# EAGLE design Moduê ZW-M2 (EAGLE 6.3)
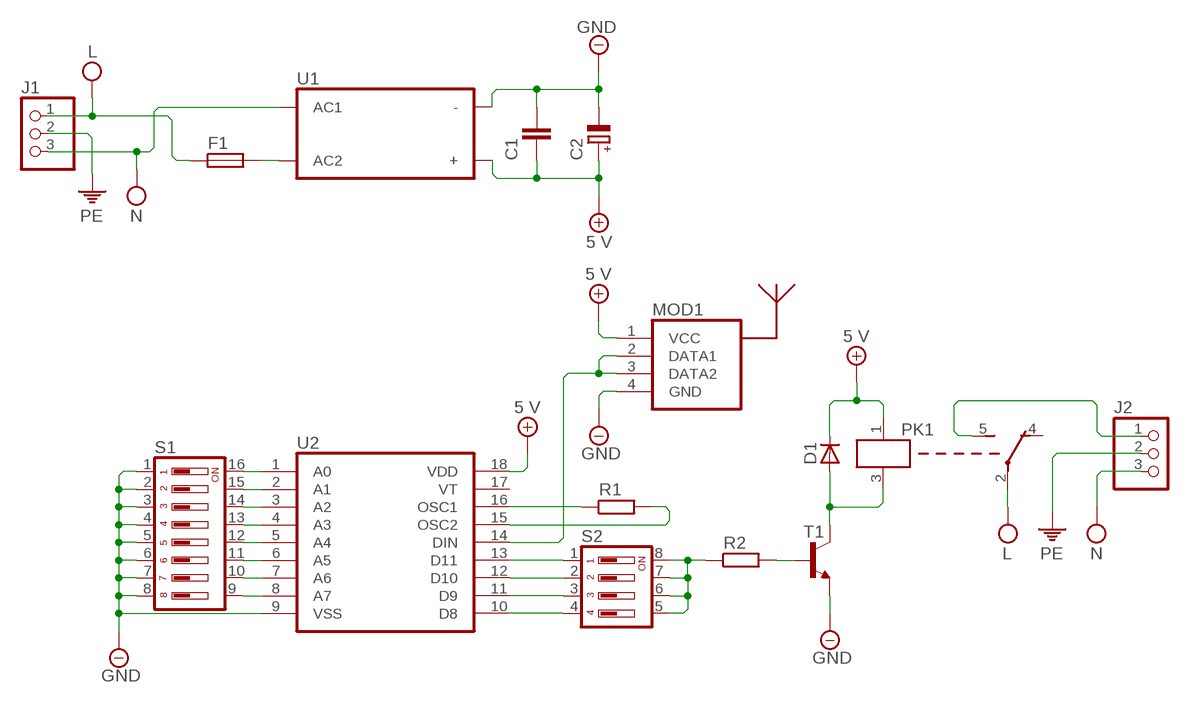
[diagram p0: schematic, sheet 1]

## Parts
C1  KONDENSATOR_CERAMICZNY  [KONDENSATOR_CERAMICZNY]
C2  KONDENSATOR_ELEKTROLITYCZNY_1  [KONDENSATOR_ELEKTROLITYCZNY_1]
D1  DIODA_PROSTOWNICZA  [DIODA_PROSTOWNICZA]
F1  BEZPIECZNIK  [BEZPIECZNIK]
J1  ZLACZE_230V  [ZLACZE_230V]
J2  ZLACZE_230V  [ZLACZE_230V]
MOD1  ODBIORNIK433MHZ  [ODBIORNIK433MHZ]
PK1  PRZEKAZNIK  [PRZEKAZNIK]
R1  REZYSTOR  [REZYSTOR]
R2  REZYSTOR  [REZYSTOR]
S1  DIP_SWITCH_8  [DIP_SWITCH_8]
S2  DIP_SWITCH_4  [DIP_SWITCH_4]
T1  TRANZYSTOR_2N3904  [TRANZYSTOR_2N3904]
U1  ZASILACZ  [ZASILACZ]
U2  HT12D  [HT12D]

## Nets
5V: C1.2 C2.+ D1.C MOD1.1(VCC) PK1.1(A1) U1.+ U2.18(VDD) ; supply symbol labelled 5 V
GND: C1.1 C2.- MOD1.4(GND) S1.1 S1.2 S1.3 S1.4 S1.5 S1.6 S1.7 S1.8 T1.E U1.- U2.9(VSS)
L: F1.1 J1.1 PK1.2(C)
N: J1.3 J2.3 U1.AC1
N$1: F1.2 U1.AC2
N$2: J2.1 PK1.5(NO)
N$3: S2.1 U2.13(D11)
N$4: S2.2 U2.12(D10)
N$5: S2.3 U2.11(D9)
N$6: S2.4 U2.10(D8)
N$7: S1.9 U2.8(A7)
N$8: R2.2 T1.B
N$9: R2.1 S2.5 S2.6 S2.7 S2.8
N$10: S1.10 U2.7(A6)
N$11: S1.11 U2.6(A5)
N$12: S1.12 U2.5(A4)
N$13: S1.13 U2.4(A3)
N$14: S1.14 U2.3(A2)
N$15: S1.15 U2.2(A1)
N$16: S1.16 U2.1(A0)
N$17: MOD1.2(DATA1) MOD1.3(DATA2) U2.14(DIN)
N$20: D1.A PK1.3(A2) T1.C
N$29: R1.2 U2.15(OSC2)
N$30: R1.1 U2.16(OSC1)
PE: J1.2 J2.2
Unconnected: PK1.4(NC) U2.17(VT)

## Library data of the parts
C1 = Własne:KONDENSATOR_CERAMICZNY
C2 = Własne:KONDENSATOR_ELEKTROLITYCZNY_1
D1 = Własne:DIODA_PROSTOWNICZA
F1 = Własne:BEZPIECZNIK
J1 J2 = Moje:ZLACZE_230V
MOD1 = Własne:ODBIORNIK433MHZ
PK1 = Moje:PRZEKAZNIK
R1 R2 = Własne:REZYSTOR
S1 = Własne:DIP_SWITCH_8
S2 = Własne:DIP_SWITCH_4
T1 = Własne:TRANZYSTOR_2N3904
U1 = Własne:ZASILACZ
U2 = Własne:HT12D

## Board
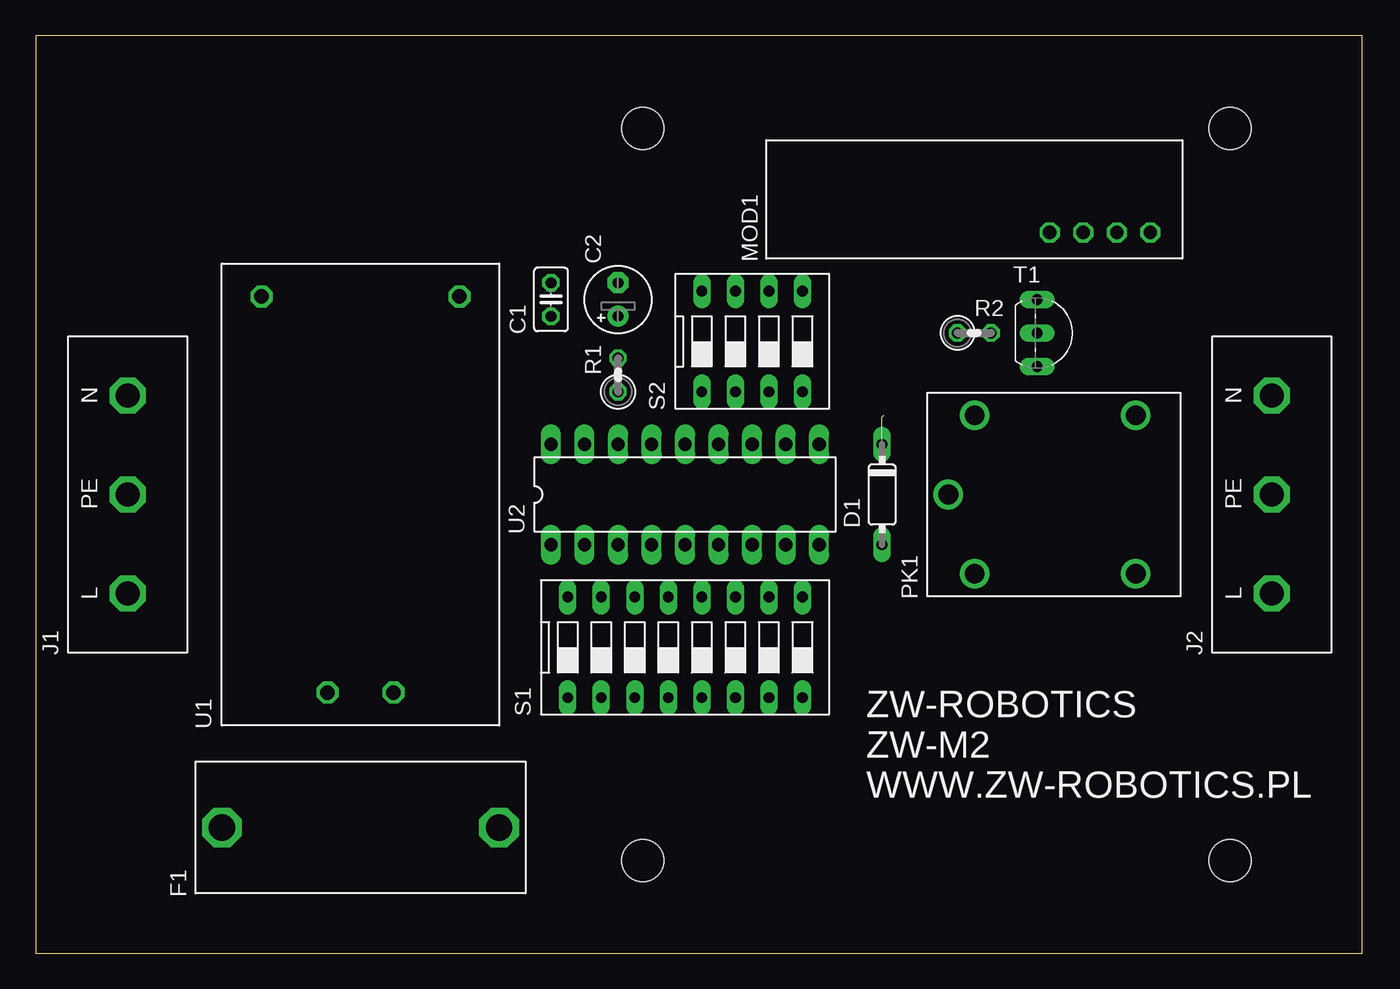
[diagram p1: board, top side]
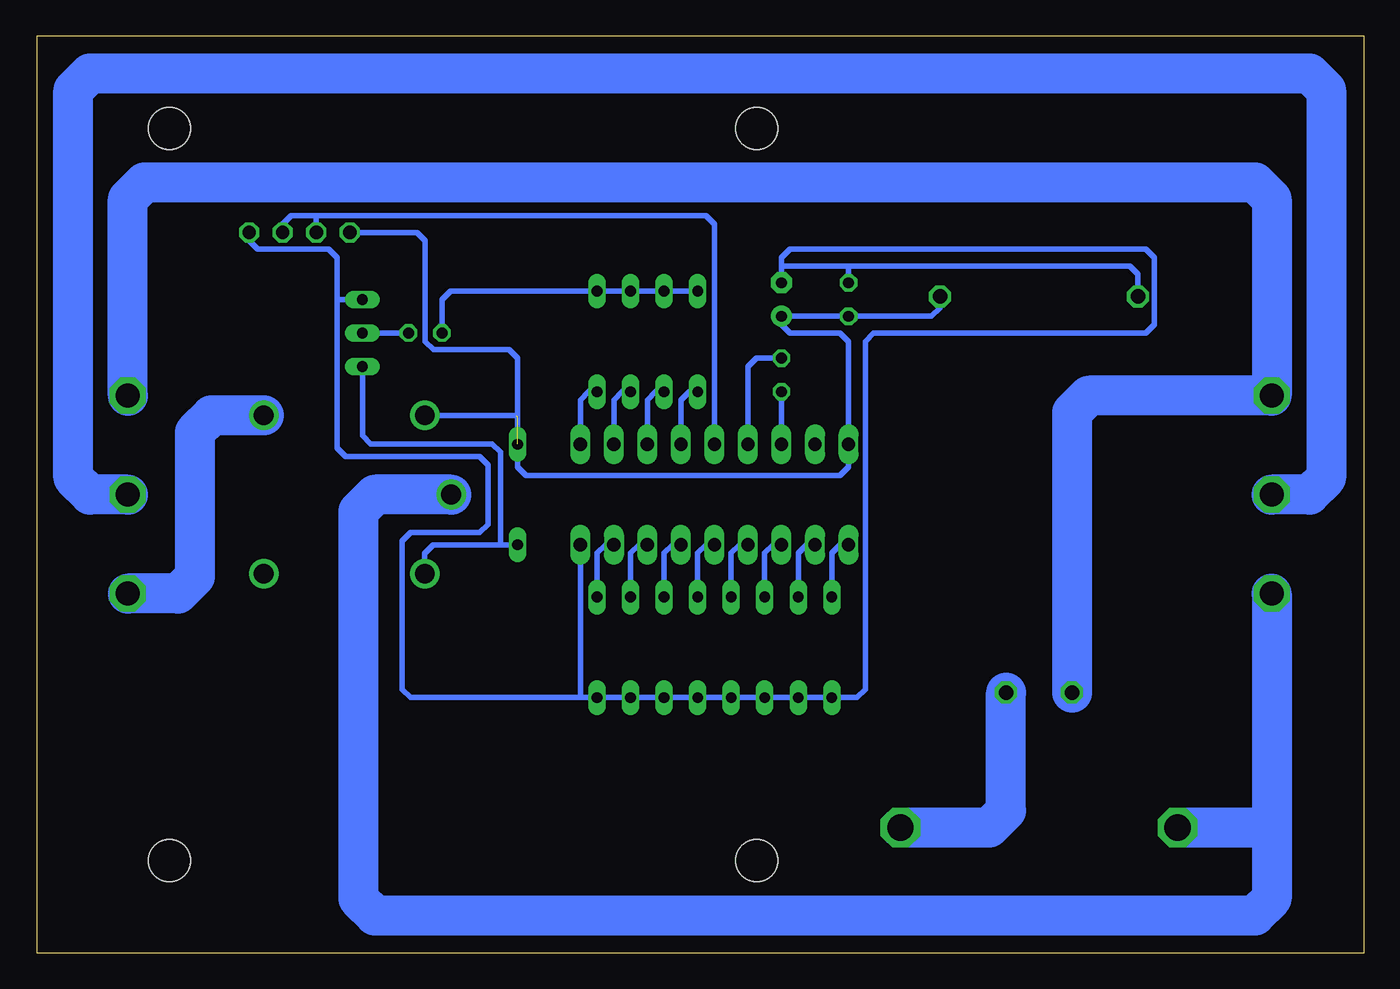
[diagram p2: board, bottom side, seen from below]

Size 100.5 x 69.5 mm. Coordinates in mm from the lower left corner, seen from the top.
Outline: 0,0 100.5,0 100.5,69.5 0,69.5 0,0
Copper layers (1*16): Top 0.035mm / dielectric 1.5mm / Bottom 0.035mm
Design rules "default": minimum track width 10mil, minimum drill 24mil, track to track 8mil, track to pad 8mil, pad to pad 8mil, via to via 8mil, smd to smd 8mil, copper to edge 40mil, drill to drill 8mil, minimum pad ring 10mil, minimum via ring 8mil, stop-mask expansion 4mil, vias tented up to drill 0mil, thermal gap 10mil
Holes 3.2 mm at 46,7 90.5,7 46,62.5 90.5,62.5

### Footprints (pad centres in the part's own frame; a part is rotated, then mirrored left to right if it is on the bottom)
KONDENSATOR_CERAMICZNY = drill 0.813 octagon: 1 -1.27,0; 2 1.27,0
KONDENSATOR_ELEKTROLITYCZNY_1 = drill 0.813 pad 1.6: + -1.27,0 | drill 0.813 pad 1.6 octagon: - 1.27,0
DIODA_PROSTOWNICZA = drill 0.813 long: A -3.81,0; C 3.81,0
BEZPIECZNIK = drill 2 octagon: 1 -10.5,0; 2 10.5,0
ZLACZE_230V = drill 1.8 octagon: 1 -7.5,0; 2 0,0; 3 7.5,0
ODBIORNIK433MHZ = drill 1 octagon: 1 -2.54,2.54; 2 -2.54,0; 3 -2.54,-2.54; 4 -2.54,-5.08
PRZEKAZNIK = drill 1.5: 1 -6,6; 2 -8,0; 3 -6,-6; 4 6.2,-6; 5 6.2,6
REZYSTOR = drill 0.813 octagon: 1 -1.27,0; 2 1.27,0
DIP_SWITCH_8 = drill 0.813 long: 1 -8.89,-3.81; 2 -6.35,-3.81; 3 -3.81,-3.81; 4 -1.27,-3.81; 5 1.27,-3.81; 6 3.81,-3.81; 7 6.35,-3.81; 8 8.89,-3.81; 9 8.89,3.81; 10 6.35,3.81; 11 3.81,3.81; 12 1.27,3.81; 13 -1.27,3.81; 14 -3.81,3.81; 15 -6.35,3.81; 16 -8.89,3.81
DIP_SWITCH_4 = drill 0.813 long: 1 -3.81,-3.81; 2 -1.27,-3.81; 3 1.27,-3.81; 4 3.81,-3.81; 5 3.81,3.81; 6 1.27,3.81; 7 -1.27,3.81; 8 -3.81,3.81
TRANZYSTOR_2N3904 = drill 0.813 long: B 0,0; C 0,-2.54; E 0,2.54
ZASILACZ = drill 1.1 octagon: + 15,-7.5; - 15,7.5; AC1 -15,2.5; AC2 -15,-2.5
HT12D = drill 1 long: 1 -10.16,-3.81; 2 -7.62,-3.81; 3 -5.08,-3.81; 4 -2.54,-3.81; 5 0,-3.81; 6 2.54,-3.81; 7 5.08,-3.81; 8 7.62,-3.81; 9 10.16,-3.81; 10 10.16,3.81; 11 7.62,3.81; 12 5.08,3.81; 13 2.54,3.81; 14 0,3.81; 15 -2.54,3.81; 16 -5.08,3.81; 17 -7.62,3.81; 18 -10.16,3.81

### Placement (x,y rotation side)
C1  39.05,49.53 270 top
C2  44.13,49.53 90 top
D1  64.14,34.75 90 top
F1  24.62,9.53 0 top
J1  6.99,34.75 90 top
J2  93.66,34.75 90 top
MOD1  79.38,57.15 90 top
PK1  77.15,34.75 0 top
R1  44.13,43.81 90 top
R2  71.12,46.99 0 top
S1  49.21,23.18 0 top
S2  54.29,46.35 0 top
T1  75.88,46.99 0 top
U1  24.62,34.75 90 top
U2  49.21,34.75 0 top

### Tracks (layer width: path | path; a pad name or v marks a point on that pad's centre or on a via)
5V  (3 unrouted)
  Bottom 0.406: 64.14,38.84 64.14,45.09 64.77,45.72 70.48,45.72 71.12,46.35 71.12,53.98 71.75,54.61 MOD1.1 | U1.+ 32.12,48.9 32.76,48.26 C1.2 C2.+ 44.13,47.62 43.5,46.99 39.69,46.99 39.05,46.35 U2.18 39.05,36.83 39.69,36.2 63.5,36.2 64.14,36.83 D1.C | PK1.1 64.25,40.75
GND
  Bottom 0.406: 77.79,49.53 77.79,52.7 78.42,53.34 83.82,53.34 84.45,53.98 MOD1.4 | 59.37,19.37 72.24,19.37 72.87,20 72.87,31.23 72.24,31.86 66.99,31.86 66.36,32.5 66.36,36.99 66.99,37.63 77.15,37.63 77.79,38.27 77.79,49.53 | 59.37,19.37 S1.8 S1.7 S1.6 S1.5 S1.4 S1.3 S1.2 S1.1 38.42,19.37 37.78,20 37.78,46.35 37.15,46.99 16.51,46.99 15.88,47.62 15.88,52.7 16.51,53.34 43.5,53.34 44.13,52.7 44.13,52.07 | T1.E 77.79,49.53 | 44.13,52.07 39.37,52.07 39.05,52.07 | 39.05,52.07 17.76,52.07 17.12,51.44 U1.- | C2.- 44.13,52.07 | U2.9 59.37,19.37 | C1.1 39.05,52.07
L
  Bottom 3.048: J1.1 6.99,9.53 | 6.99,9.53 6.99,4.13 8.26,2.86 74.93,2.86 76.2,4.13 76.2,33.48 74.93,34.75 PK1.2 | F1.1 6.99,9.53
N
  Bottom 3.048: U1.AC1 22.12,40.98 20.85,42.25 J1.3 6.99,57.15 8.26,58.42 92.39,58.42 93.66,57.15 J2.3
N$1
  Bottom 3.048: F1.2 28.39,9.53 27.12,10.79 U1.AC2
N$2
  Bottom 3.048: J2.1 89.85,27.25 88.58,28.52 88.58,39.48 87.31,40.75 PK1.5
N$3
  Bottom 0.406: U2.13 51.75,41.91 51.12,42.55 S2.1
N$4
  Bottom 0.406: U2.12 54.29,41.91 53.66,42.55 S2.2
N$5
  Bottom 0.406: U2.11 56.83,41.91 56.2,42.55 S2.3
N$6
  Bottom 0.406: U2.10 59.37,41.91 58.74,42.55 S2.4
N$7
  Bottom 0.406: S1.9 58.1,30.3 57.47,30.94 U2.8
N$8
  Bottom 0.406: R2.2 T1.B
N$9
  Bottom 0.406: S2.8 S2.7 S2.6 S2.5 69.22,50.16 69.85,49.53 R2.1
N$10
  Bottom 0.406: S1.10 55.56,30.3 54.93,30.94 U2.7
N$11
  Bottom 0.406: S1.11 53.02,30.3 52.39,30.94 U2.6
N$12
  Bottom 0.406: S1.12 50.48,30.3 49.85,30.94 U2.5
N$13
  Bottom 0.406: S1.13 47.94,30.3 47.31,30.94 U2.4
N$14
  Bottom 0.406: S1.14 45.4,30.3 44.77,30.94 U2.3
N$15
  Bottom 0.406: S1.15 42.86,30.3 42.23,30.94 U2.2
N$16
  Bottom 0.406: S1.16 40.32,30.3 39.69,30.94 U2.1
N$17
  Bottom 0.406: U2.14 49.21,55.24 49.85,55.88 79.38,55.88 | 79.38,55.88 MOD1.2 | MOD1.3 81.92,55.24 81.28,55.88 79.38,55.88
N$20
  Bottom 0.406: 65.41,30.91 65.41,37.96 66.04,38.59 75.25,38.59 75.88,39.23 T1.C | 65.41,30.91 70.52,30.91 71.15,30.28 PK1.3 | 65.41,30.91 64.16,30.91
  Bottom 0.61: 64.16,30.91 D1.A
N$29
  Bottom 0.406: U2.15 46.67,44.45 46.04,45.09 R1.2
N$30
  Bottom 0.406: U2.16 R1.1
PE
  Bottom 3.048: J1.2 4.13,34.75 2.86,36.02 2.86,65.41 4.13,66.67 96.52,66.67 97.79,65.41 97.79,36.02 96.52,34.75 J2.2

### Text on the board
tNames: ZW-ROBOTICS / ZW-M2 / WWW.ZW-ROBOTICS.PL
